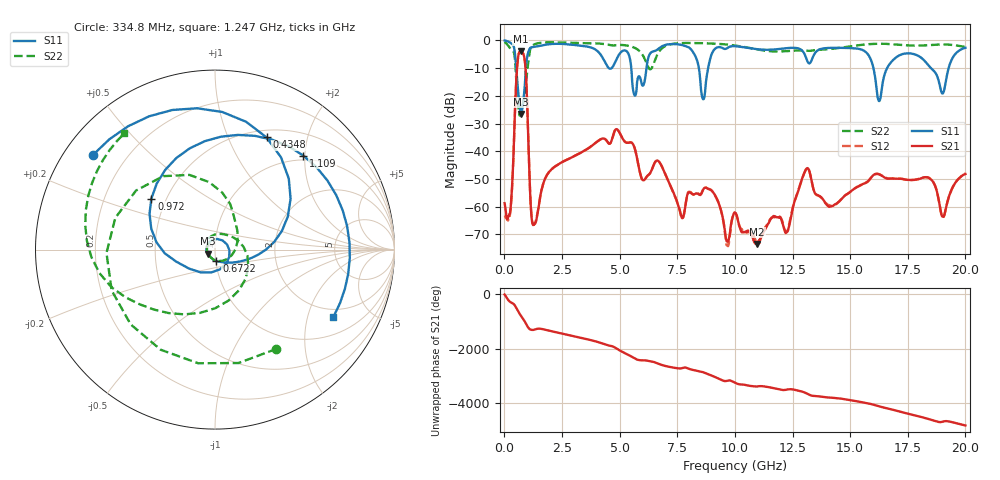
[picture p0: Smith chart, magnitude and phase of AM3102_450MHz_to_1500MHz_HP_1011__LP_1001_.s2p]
!Agilent Technologies,E8364B,MY43040894,A.07.50.67
!Agilent E8364B: A.07.50.67
!Date: Thursday, January 11, 2018 06:25:17
!Correction: S11(Full 2 Port(1,2))
!S21(Full 2 Port(1,2))
!S12(Full 2 Port(1,2))
!S22(Full 2 Port(1,2))
!S2P File: Measurements: S11, S21, S12, S22:
# Hz S  dB  R 50
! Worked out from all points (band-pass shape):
!   1601 points, 10 MHz to 20 GHz, reference 50 ohm
!   highest |S21| = -3.93 dB at 709.6 MHz (marker M1); lowest = -73.4 dB at 10.97 GHz (marker M2)
!   |S21| within 3 dB of the highest: 581.9 MHz to 880.2 MHz (298.3 MHz wide, 40.8 % of centre)
!   lowest |S11| = -26.5 dB at 722.1 MHz (marker M3), VSWR 1.10, Z = 46 - j2.01 ohm
!   |S11| at or under -10 dB: 5.506 GHz to 6.165 GHz (659.1 MHz wide, 11.3 % of centre); 16.01 GHz to 16.6 GHz (593.6 MHz wide, 3.64 % of centre); 18.5 GHz to 19.27 GHz (771 MHz wide, 4.08 % of centre)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
!   |S22| runs from -27.1 to -0.6 dB; largest |S21 - S12| = 0.0007
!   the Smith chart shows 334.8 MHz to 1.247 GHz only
!   S11 on the Smith chart (normalised r, x): 334.8 MHz: 0.08, +0.34; 434.8 MHz: 0.59, +1.39; 672.2 MHz: 1.01, -0.13; 972 MHz: 0.41, +0.30; 1.109 GHz: 0.91, +1.97; 1.247 GHz: 1.66, -2.93
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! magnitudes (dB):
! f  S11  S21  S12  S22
! 10 MHz  -0.1  -58.7  -63.1  -0.6
! 334.8 MHz  -1.3  -52.5  -53.0  -3.7
! 434.8 MHz  -3.2  -31.5  -31.6  -5.2
! 672.2 MHz  -23.8  -4.1  -4.1  -27.1
! 709.6 MHz  -26.4  -3.9  -3.9  -26.5
! 722.1 MHz  -26.5  -3.9  -3.9  -25.7
! 972 MHz  -6.8  -19.0  -19.0  -12.6
! 1.109 GHz  -2.9  -53.5  -53.3  -3.7
! 1.247 GHz  -2.4  -66.6  -66.2  -1.7
! 3.346 GHz  -2.0  -40.4  -40.4  -1.0
! 5.657 GHz  -19.9  -39.0  -39.0  -2.7
! 6.682 GHz  -3.1  -43.5  -43.5  -4.4
! 7.694 GHz  -1.7  -63.9  -64.1  -1.0
! 8.618 GHz  -21.2  -53.9  -53.8  -1.0
! 9.668 GHz  -2.8  -72.5  -74.1  -1.5
! 10.01 GHz  -2.1  -62.2  -62.2  -1.9
! 10.97 GHz  -3.2  -73.4  -73.3  -3.3
! 13.34 GHz  -6.9  -51.3  -51.2  -3.7
! 16.25 GHz  -21.9  -48.3  -48.2  -1.2
! 16.68 GHz  -9.0  -49.9  -49.9  -1.3
! 19.03 GHz  -19.1  -63.6  -63.8  -1.5
! 20 GHz  -2.7  -48.2  -48.0  -2.3
